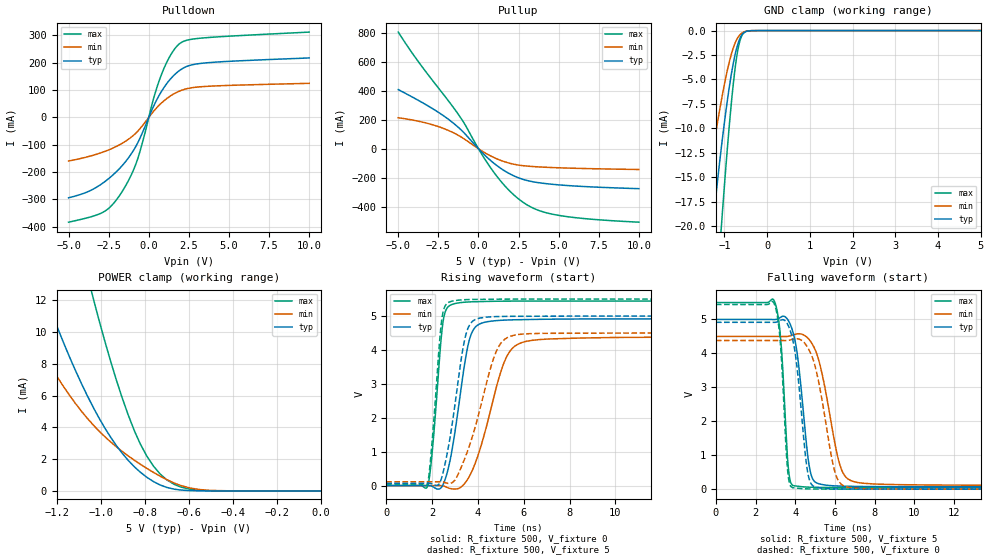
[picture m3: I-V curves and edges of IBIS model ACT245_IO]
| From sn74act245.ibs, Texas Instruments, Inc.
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[Model]   ACT245_IO
Model_type  I/O
Vinl = 0.8
Vinh = 2
Enable   Active-Low
Vref =   0
Rref =   500
Cref =   50p
Vmeas =   1.5
| variable   typ   min   max
C_comp   6.88pF   6.27pF   7.73pF
| C_pullup   12.46pF   7.19pF   18.22pF
| C_pulldown   8.70pF   7.22pF   10.91pF
| C_tri-state   6.88pF   6.27pF   7.73pF
[Temperature Range]   40   100   -40
| Ambient temperature   25   85   -40
[Voltage range]   5   4.5   5.5
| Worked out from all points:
|   slope of the pulldown table from 0 to 0.75 V, typ, clamps not added: 8.23 ohm
|   slope of the pullup table from 0 to 0.75 V, typ, clamps not added: 9.31 ohm
|   GND clamp passes 1 mA (typ) near -0.66 V on its own axis
|   POWER clamp passes 1 mA (typ) near -0.80 V on its own axis
|   rising waveform, R_fixture 500, V_fixture 0: 20-80 % time 656ps typ, 1.08ns min, 380ps max; typ from 0 V to 4.92 V
|   falling waveform, R_fixture 500, V_fixture 5: 20-80 % time 524ps typ, 863ps min, 320ps max; typ from 5 V to 0.068 V
|   rising waveform, R_fixture 500, V_fixture 5: 20-80 % time 651ps typ, 1.09ns min, 366ps max; typ from 0.068 V to 5 V
|   falling waveform, R_fixture 500, V_fixture 0: 20-80 % time 499ps typ, 801ps min, 308ps max; typ from 4.92 V to 0 V
[GND Clamp]
| ACT245_IO
|   Voltage   I(typ)   I(min)   I(max)
-5V       -257.6mA   -168.5mA   -326.6mA
-1.555V   -33mA      -20.85mA   -52.14mA
-1.505V   -30.55mA   -19.27mA   -48.61mA
-1.3V     -21.11mA   -13.12mA   -34.54mA
-1.25V    -18.97mA   -11.72mA   -31.23mA
-1.075V   -12.02mA   -7.192mA   -20.19mA
-1.055V   -11.29mA   -6.717mA   -18.99mA
-895mV    -6.015mA   -3.35mA    -10.12mA
-765mV    -2.74mA    -1.424mA   -4.358mA
-665mV    -1.098mA   -573.1uA   -1.518mA
-545mV    -209.6uA   -135.1uA   -215.6uA
5V        95.62nA    30.48uA    872nA
[POWER Clamp]
| ACT245_IO
|   Voltage   I(typ)   I(min)   I(max)
-5V       307.3mA    212.4mA    474.5mA
-1.41V    18.74mA    12.56mA    36.85mA
-1.38V    17.45mA    11.72mA    34.58mA
-1.26V    12.61mA    8.625mA    25.99mA
-1.06V    5.976mA    4.561mA    13.55mA
-1.03V    5.163mA    4.094mA    11.92mA
-930mV    2.876mA    2.792mA    7.033mA
-845mV    1.49mA     1.91mA     3.717mA
-790mV    853uA      1.412mA    2.173mA
-700mV    219.2uA    708.8uA    695.5uA
-550mV    5.632uA    85.11uA    35.96uA
-84.45fV  95.62nA    5.578nA    1.326uA
[Pulldown]
| ACT245_IO
|   Voltage   I(typ)   I(min)   I(max)
-5V       -293.7mA   -159.3mA   -383mA
-3.775V   -271mA     -143.3mA   -366mA
-2.79V    -236.8mA   -125.3mA   -344.4mA
-2.24V    -210.6mA   -112.1mA   -317.2mA
-1.62V    -173.6mA   -93.21mA   -267.2mA
-700mV    -94.19mA   -51.12mA   -153mA
310mV     42.12mA    23.14mA    71.14mA
790mV     94.99mA    52.74mA    156.8mA
1.355V    140.8mA    78.81mA    227.4mA
1.915V    171.6mA    96.32mA    269.6mA
3.475V    199.1mA    113.2mA    291.2mA
10V       217.6mA    124.7mA    312.1mA
[Pullup]
| ACT245_IO
|   Voltage   I(typ)   I(min)   I(max)
-5V       407.1mA    213.1mA    803.2mA
-3.73V    331.9mA    189mA      596.8mA
-1.745V   191.9mA    119.5mA    311mA
-935mV    113.5mA    70.59mA    183.3mA
120mV     -14.11mA   -8.809mA   -22.35mA
885mV     -93.23mA   -56.6mA    -151.2mA
1.7V      -157.3mA   -92.23mA   -262.6mA
2.515V    -201.2mA   -113mA     -347.1mA
3.52V     -229.9mA   -123.7mA   -414.7mA
4.755V    -246.6mA   -130.4mA   -454.1mA
6.77V     -261.5mA   -136.8mA   -482.8mA
10V       -275.1mA   -143.1mA   -506mA
[Ramp]
| ACT245_IO
| variable   typ   min   max
dV/dt_r   3.01/6.74E-10   2.69/1.11E-09   3.31/3.86E-10
dV/dt_f   3.02/5.43E-10   2.68/8.84E-10   3.33/3.35E-10
R_load = 500
[Rising Waveform]
| ACT245_IO
R_fixture =   500
C_fixture =   0
L_fixture =   0
V_fixture =   0
V_fixture_min = 0
V_fixture_max = 0
|   Time   V(typ)   V(min)   V(max)
0s        32.92nV    7.046nV    244.4nV
1.81ns    1.25mV     -62.17uV   -11.78mV
2.01ns    -23.21mV   -111.9uV   1.02V
2.49ns    45.08mV    -10.36mV   4.873V
3.145ns   2.265V     -86.67mV   5.386V
3.54ns    4.043V     172.4mV    5.413V
3.87ns    4.659V     635.4mV    5.422V
5.215ns   4.881V     3.744V     5.439V
6.34ns    4.898V     4.281V     5.441V
50ns      4.917V     4.381V     5.442V
[Falling Waveform]
| ACT245_IO
R_fixture =   500
C_fixture =   0
L_fixture =   0
V_fixture =   5
V_fixture_min = 4.5
V_fixture_max = 5.5
|   Time   V(typ)   V(min)   V(max)
0s        5V         4.5V       5.5V
2.955ns   4.999V     4.5V       5.526V
3.27ns    5.069V     4.5V       4.375V
3.66ns    4.957V     4.505V     559.5mV
3.96ns    4.446V     4.558V     97.46mV
4.735ns   575.5mV    4.379V     58.31mV
5.44ns    127.4mV    3.148V     50.3mV
6.31ns    90.08mV    605.5mV    46.64mV
7.365ns   79.2mV     177.4mV    44.96mV
50ns      68.27mV    112.4mV    43.77mV
[Rising Waveform]
| ACT245_IO
R_fixture =   500
C_fixture =   0
L_fixture =   0
V_fixture =   5
V_fixture_min = 4.5
V_fixture_max = 5.5
|   Time   V(typ)   V(min)   V(max)
0s        68.27mV    112.4mV    43.77mV
1.79ns    69.24mV    112.4mV    39.79mV
1.96ns    60.33mV    112.3mV    966.7mV
2.435ns   268.8mV    110mV      4.949V
3ns       2.394V     165.6mV    5.455V
3.385ns   4.178V     726.7mV    5.48V
3.68ns    4.782V     1.278V     5.488V
4.81ns    4.983V     3.968V     5.496V
5.755ns   4.992V     4.454V     5.499V
50ns      5V         4.5V       5.5V
[Falling Waveform]
| ACT245_IO
R_fixture =   500
C_fixture =   0
L_fixture =   0
V_fixture =   0
V_fixture_min = 0
V_fixture_max = 0
|   Time   V(typ)   V(min)   V(max)
0s        4.917V     4.381V     5.442V
2.94ns    4.915V     4.381V     5.464V
3.235ns   4.969V     4.38V      4.387V
3.62ns    4.85V      4.382V     505.9mV
3.87ns    4.402V     4.416V     42.41mV
4.625ns   493.3mV    4.173V     8.899mV
5.19ns    41.65mV    3.124V     3.627mV
6.025ns   7.767mV    452.1mV    1.345mV
6.89ns    2.81mV     34.24mV    597.8uV
50ns      29.84nV    9.861nV    241.4nV
